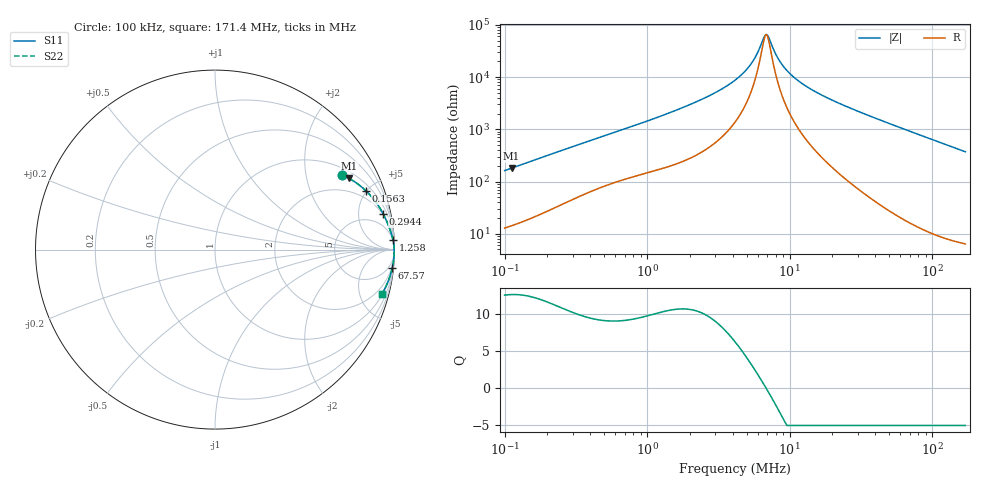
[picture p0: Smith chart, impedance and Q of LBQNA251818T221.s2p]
! LBQNA251818T221  S-PARAMETER MODEL  ( General Type )
! Model Generated by TAIYO YUDEN Corporation (http://www.ty-top.com)
! Version 1.0
! TAIYO YUDEN Control No. 191025NI43SB-FBB
! Copyright(c) 2019 TAIYO YUDEN CO.,LTD. All Rights Reserved.
! Product Description (link to TY-COMPAS)
! https://ds.yuden.co.jp/TYCOMPAS/or/detail?pn=LBQNA251818T221K&u=M
! Products Name : Inductors
! Characteristics :
!  Inductance : 220 uH , SRF(min) : 5.5 MHz , DC Resistance(max) : 5.85 Ohm
!  Rated Current : Saturation :50 mA , Temp Rise : 110 mA (20 degC)
!  Case Size : 2.5 x 1.8 / 0.098 x 0.071 [mm/inch] , Thickness : 1.8 / 0.071 [mm/inch]
!  (Conditions: Temperature = 25 degC , DC Bias Current/Voltage = 0A / 0V)
! External Node Assignments :
!  1  o---GGG---o  2
! GND o---------o GND
! Frequency Range : 0.1MHz  -  171.398534MHz  [ 402 STEP ]
# MHz S RI R 50
! Freq[MHz].  S11 Real  S11 Imag  S21 Real  S21 Imag  S12 Real  S12 Imag  S22 Real  S22 Imag
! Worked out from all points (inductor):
!   401 points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, 100 kHz to 171.4 MHz, reference 50 ohm
!   read as one part in series: L = 254 uH near 103.8 kHz
!   highest Q = 12.7 at 111.8 kHz (marker M1), where L = 256 uH
!   self-resonance near 6.844 MHz
!   S11 on the Smith chart (normalised r, x): 100 kHz: 1.26, +3.22; 156.3 kHz: 1.40, +4.97; 294.4 kHz: 1.88, +9.09; 1.258 MHz: 4, +36; 67.57 MHz: 1, -19; 171.4 MHz: 1.13, -7.41
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0.1  0.7083 0.4165  0.2917 -0.4165  0.2917 -0.4165  0.7083 0.4165
0.111818  0.7479 0.3965  0.2521 -0.3965  0.2521 -0.3965  0.7479 0.3965
0.156329  0.8424 0.3261  0.1576 -0.3261  0.1576 -0.3261  0.8424 0.3261
0.294395  0.9366 0.1999  0.0634 -0.1999  0.0634 -0.1999  0.9366 0.1999
0.348094  0.9496 0.1736  0.0504 -0.1736  0.0504 -0.1736  0.9496 0.1736
1.211692  0.9912 0.0565  0.00881 -0.0565  0.00881 -0.0565  0.9912 0.0565
1.257658  0.9917 0.0545  0.00833 -0.0545  0.00833 -0.0545  0.9917 0.0545
2.59943  0.997 0.0241  0.00303 -0.0241  0.00303 -0.0241  0.997 0.0241
4.140031  0.9981 0.0113  0.00193 -0.0113  0.00193 -0.0113  0.9981 0.0113
5.372715  0.9983 0.00531  0.00165 -0.00531  0.00165 -0.00531  0.9983 0.00531
5.896834  0.9984 0.00327  0.00159 -0.00327  0.00159 -0.00327  0.9984 0.00327
6.593697  0.9985 0.00085  0.00154 -0.00085  0.00154 -0.00085  0.9985 0.00085
6.843827  0.9985 4.84e-05  0.00153 -4.84e-05  0.00153 -4.84e-05  0.9985 4.84e-05
7.103446  0.9985 -0.000754  0.00152 0.000754  0.00152 0.000754  0.9985 -0.000754
8.399129  0.9985 -0.00439  0.00149 0.00439  0.00149 0.00439  0.9985 -0.00439
9.391703  0.9985 -0.00688  0.0015 0.00688  0.0015 0.00688  0.9985 -0.00688
11.31344  0.9984 -0.0112  0.00156 0.0112  0.00156 0.0112  0.9984 -0.0112
14.41119  0.9983 -0.0175  0.00173 0.0175  0.00173 0.0175  0.9983 -0.0175
23.38354  0.9974 -0.0336  0.00256 0.0336  0.00256 0.0336  0.9974 -0.0336
50.16444  0.9924 -0.0769  0.0076 0.0769  0.0076 0.0769  0.9924 -0.0769
67.57036  0.9872 -0.1039  0.0128 0.1039  0.0128 0.1039  0.9872 -0.1039
171.3985  0.9284 -0.2493  0.0716 0.2493  0.0716 0.2493  0.9284 -0.2493
